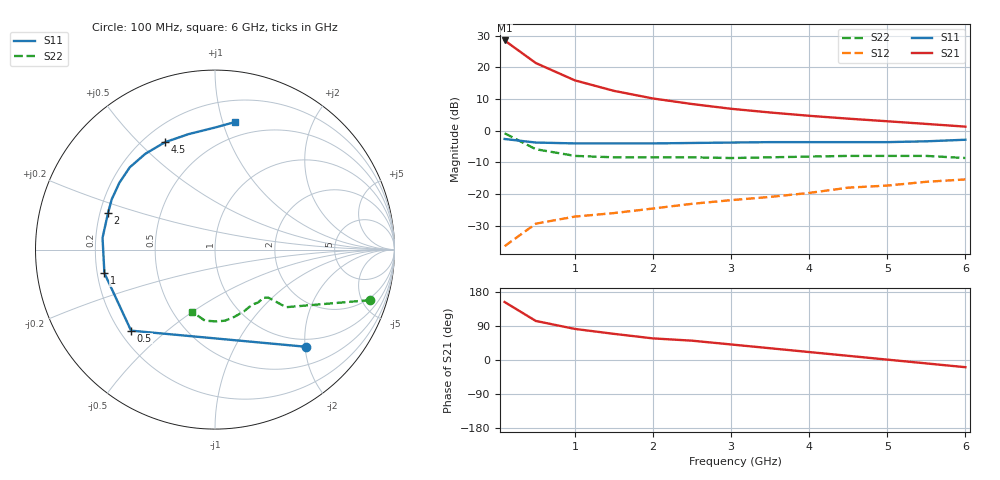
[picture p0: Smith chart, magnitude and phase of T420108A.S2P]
!AT-42010
!S AND NOISE PARAMETERS at Vce=8V  Ic=10mA.  LAST UPDATED 07-21-92
# ghz s ma r 50
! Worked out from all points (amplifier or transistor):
!   13 points, 100 MHz to 6 GHz, reference 50 ohm
!   highest |S21| = 28.5 dB at 100 MHz (marker M1)
!   |S21| within 3 dB of that: start of sweep to 268 MHz
!   unconditionally stable (mu >= 1): 1.329 GHz to 5.564 GHz
!   at 1 GHz: K = 0.85, MSG = 21.5 dB, |S12| = -27.1 dB
!   at 3 GHz: K = 1.25, MAG = 11.4 dB, |S12| = -21.9 dB
!   at 6 GHz: K = 0.95, MSG = 8.3 dB, |S12| = -15.4 dB
!   lowest NFmin = 1.00 dB at 100 MHz
!   S11 on the Smith chart (normalised r, x): 100 MHz: 0.84, -2.01; 500 MHz: 0.24, -0.38; 1 GHz: 0.23, -0.10; 2 GHz: 0.23, +0.16; 4.5 GHz: 0.28, +0.60; 6 GHz: 0.37, +1.10
0.1  0.74 -47.0  26.65 153.0  0.015 72.0  0.91 -18.0
0.5  0.65 -136.0  11.71 103.0  0.034 38.0  0.51 -39.0
1  0.63 -168.0  6.24 82.0  0.044 36.0  0.4 -42.0
1.5  0.63 174.0  4.26 69.0  0.05 42.0  0.38 -45.0
2  0.63 161.0  3.23 57.0  0.059 43.0  0.38 -49.0
2.5  0.64 154.0  2.64 51.0  0.07 52.0  0.38 -51.0
3  0.65 145.0  2.22 41.0  0.08 54.0  0.37 -56.0
3.5  0.66 136.0  1.94 31.0  0.09 51.0  0.38 -65.0
4  0.66 126.0  1.72 21.0  0.104 50.0  0.39 -74.0
4.5  0.66 115.0  1.55 11.0  0.126 45.0  0.4 -82.0
5  0.66 103.0  1.41 1.0  0.136 41.0  0.4 -89.0
5.5  0.68 90.0  1.28 -9.0  0.156 36.0  0.4 -98.0
6  0.72 81.0  1.16 -19.0  0.17 31.0  0.37 -110.0
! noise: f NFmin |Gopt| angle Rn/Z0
0.1  1  0.04  15  0.13
0.5  1.1  0.05  76  0.12
1  1.5  0.1  132  0.12
2  1.9  0.23  -177  0.11
4  3  0.45  -125  0.26
